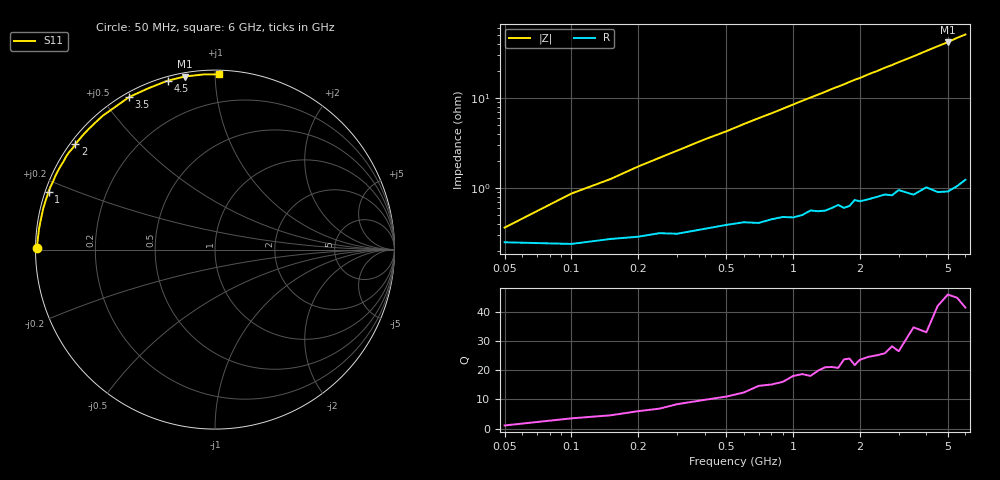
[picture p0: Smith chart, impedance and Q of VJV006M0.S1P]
! Infineon Technologies  Discrete & RF Semiconductors
! BB 914
! Si Tuning Diode in SOT23
! VR =
! S-Parameters:  July  1999
# GHz  S  MA  R  50
!  f  S11
! GHz  MAG  ANG
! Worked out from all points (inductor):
!   34 points, 50 MHz to 6 GHz, reference 50 ohm
!   read as one part to ground: L = 1.32 nH near 100 MHz
!   highest Q = 45 at 5 GHz (marker M1), where L = 1.34 nH
!   S11 on the Smith chart (normalised r, x): 50 MHz: 0.00, +0.01; 1 GHz: 0.01, +0.17; 2 GHz: 0.01, +0.33; 3.5 GHz: 0.02, +0.58; 4.5 GHz: 0.02, +0.76; 6 GHz: 0.02, +1.02
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0.05  0.9902 179.4
0.1  0.9906 178.1
0.15  0.9893 177.2
0.2  0.9887 176.1
0.4  0.9862 172.1
0.5  0.9848 170.3
0.7  0.9841 166.4
0.8  0.9826 164.6
1  0.982 160.8
1.1  0.981 158.9
1.4  0.9791 153.5
1.5  0.9778 151.6
1.6  0.9763 149.9
1.7  0.9781 148.2
1.8  0.9772 146.3
1.9  0.9738 144.5
2  0.9749 143.0
2.2  0.974 139.4
2.4  0.973 136.3
2.6  0.9721 132.8
2.8  0.9733 129.9
3  0.9703 126.6
3.5  0.9753 119.4
4  0.9725 112.2
4.5  0.9775 105.7
5  0.9789 99.9
5.5  0.9781 93.6
6  0.9763 88.6
